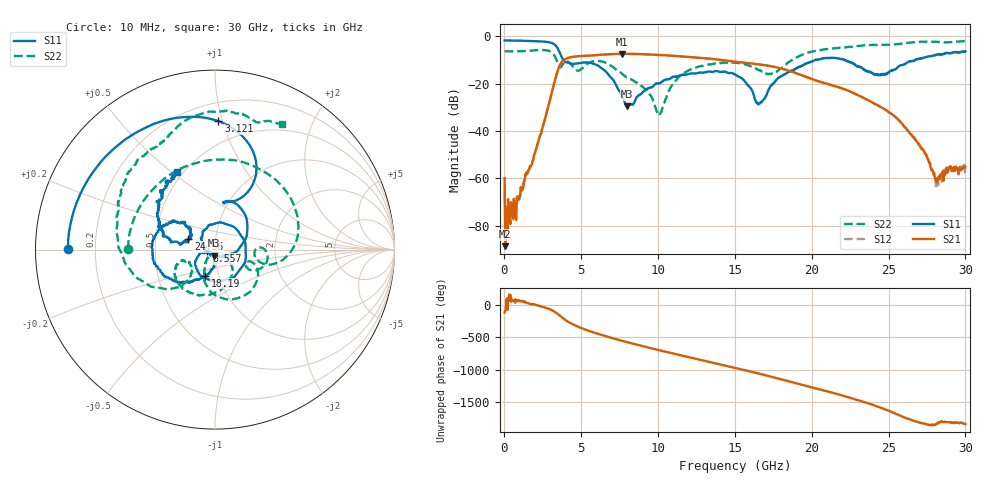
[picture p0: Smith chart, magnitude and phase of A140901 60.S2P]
!  2-Port S-parameters saved by WinCal
! VAR MeasName=S-Parameters (CALIBRATED_DATA) read from VNA (N5244A)
! VAR MeasDate=11/3/2014 9:36:37 AM
! VAR NAME=A140901 60
! VAR FILENAME=A140901 60.S2P
! VAR DATE=11/3/2014 9:36:37 AM
! VAR PHYS_PORTS=1,2
# Hz S RI R 50
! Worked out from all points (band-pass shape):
!   801 points, 10 MHz to 30 GHz, reference 50 ohm
!   highest |S21| = -7.39 dB at 7.657 GHz (marker M1); lowest = -88.7 dB at 47.49 MHz (marker M2)
!   |S21| within 3 dB of the highest: 3.787 GHz to 14.67 GHz (10.89 GHz wide, 118 % of centre)
!   lowest |S11| = -29.5 dB at 7.995 GHz (marker M3), VSWR 1.07, Z = 49.5 - j3.3 ohm
!   |S11| at or under -10 dB: 3.83 GHz to 20.23 GHz (16.4 GHz wide, 136 % of centre); 22.12505 GHz to 22.13837 GHz (13.32 MHz wide, 0.0602 % of centre); 22.18 GHz to 26.73 GHz (4.551 GHz wide, 18.6 % of centre)
!   |S22| runs from -33.2 to -2.0 dB; largest |S21 - S12| = 0.0022
!   S11 on the Smith chart (normalised r, x): 10 MHz: 0.10, +0.00; 3.121 GHz: 0.33, +0.97; 8.557 GHz: 0.91, -0.01; 18.19 GHz: 0.86, -0.26; 24.56 GHz: 0.74, +0.09; 30 GHz: 0.47, +0.52
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1e7  -0.8177 0.00171  -0.000399 -0.000925  0.000303 -0.000377  -0.4846 0.00415
4.74875e7  -0.8189 0.015  3.55e-06 -3.67e-05  0.000144 -0.000213  -0.4835 0.0211
1.974375e8  -0.8171 0.064  2.77e-05 -7.95e-05  -0.000221 2.32e-05  -0.4766 0.0884
8.722125e8  -0.7634 0.279  0.000185 0.000352  0.000235 0.000356  -0.3394 0.3427
2.071812e9  -0.5033 0.6113  0.00425 -2.28e-05  0.00415 0.000108  0.1563 0.4876
3.121462e9  0.0185 0.7158  0.00935 -0.0725  0.00933 -0.0723  0.4437 0.0259
3.833725e9  0.137 0.2835  -0.2759 0.1461  -0.2758 0.1459  0.2676 0.00803
5.033325e9  0.0623 0.2693  0.3842 0.0174  0.384 0.0175  0.1973 -0.0666
6.270412e9  0.1804 0.1225  -0.0481 -0.4063  -0.0477 -0.4055  0.1199 -0.2727
7.65745e9  0.0383 -0.0398  -0.4183 0.0856  -0.4178 0.0849  -0.0616 -0.1486
7.994838e9  -0.0035 -0.0333  -0.3582 0.2315  -0.3583 0.2306  -0.0598 -0.1218
8.55715e9  -0.0472 -0.00775  -0.1621 0.3924  -0.1631 0.3922  -0.0563 -0.0908
1.001916e10  -0.0765 0.0671  0.364 0.182  0.3634 0.1819  -0.00545 -0.0222
1.208098e10  0.1011 0.128  0.00959 -0.3648  0.01 -0.3642  0.0763 -0.1826
1.5005e10  -0.0939 -0.1245  -0.1016 0.2742  -0.1008 0.2739  -0.2019 -0.1908
1.654199e10  -0.0325 -0.0193  0.2342 0.1029  0.2344 0.1034  -0.1829 -0.062
1.819144e10  -0.0553 -0.1454  0.0415 -0.197  0.0418 -0.1974  -0.1555 -0.1768
2.002832e10  -0.2481 -0.1624  -0.1221 0.0255  -0.1225 0.0249  -0.4563 -0.1345
2.456431e10  -0.1492 0.0589  -0.0269 -0.016  -0.0267 -0.0161  -0.3551 0.5591
2.501416e10  -0.1634 0.0436  -0.0246 0.00495  -0.0249 0.00489  -0.3018 0.5947
2.816311e10  -0.3155 0.2683  0.00073 -0.000361  0.000691 -0.000153  0.1643 0.75
3e10  -0.2099 0.4298  0.00139 -0.00106  0.00135 -0.000948  0.374 0.7009
